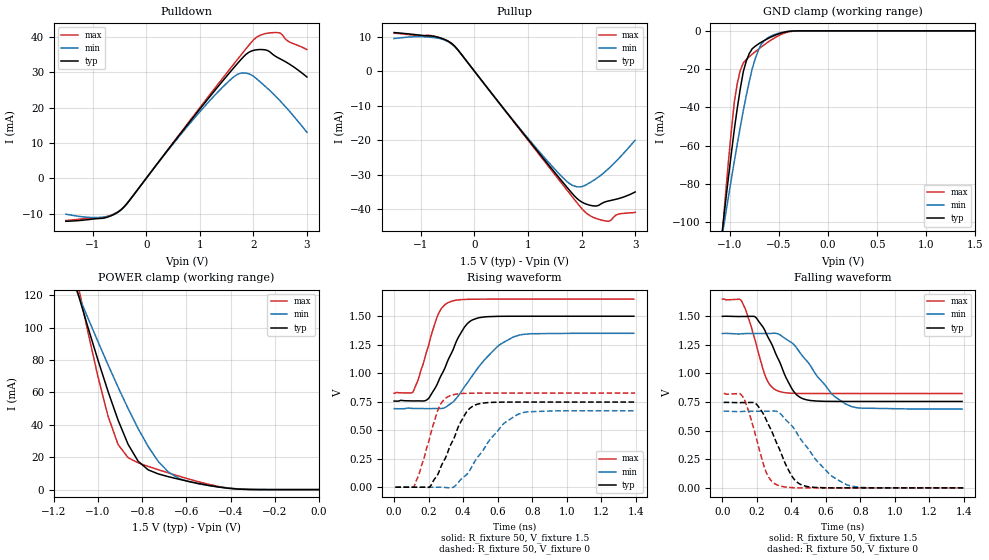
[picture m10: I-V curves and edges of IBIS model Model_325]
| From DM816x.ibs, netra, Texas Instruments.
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| Model based on original model for BSHTLTCSCDDVGPBFZ
|   Sub model SLOWEST_8MA_10PER_N_1P5
[model]   Model_325
|[Description]  1.5V-3-STATE-X-SLOWEST, 8MA, +-10%
|[Input Load]
|[Output Drive] SLOWEST, 8MA
|Voltage   1.5V
|Mode   3-STATE
Model_type   3-state
Polarity   Non-Inverting
Enable   Active-Low
Cref =  15.0000pF
Rref =  100.0000M
Vref =  0V
Vmeas =  0.75
C_comp   1.5249p   1.4275p   1.6205p
[Model Spec]
[Temperature Range]   25   125   -40
[Voltage Range]   1.5   1.35   1.65
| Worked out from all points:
|   slope of the pulldown table from 0 to 0.225 V, typ, clamps not added: 50.1 ohm
|   slope of the pullup table from 0 to 0.225 V, typ, clamps not added: 50.1 ohm
|   GND clamp passes 1 mA (typ) near -0.47 V on its own axis
|   POWER clamp passes 1 mA (typ) near -0.42 V on its own axis
|   rising waveform, R_fixture 50, V_fixture 1.5: 20-80 % time 136ps typ, 207ps min, 98.7ps max; typ from 0.756 V to 1.5 V
|   rising waveform, R_fixture 50, V_fixture 0: 20-80 % time 132ps typ, 190ps min, 95.7ps max; typ from 0 V to 0.747 V
|   falling waveform, R_fixture 50, V_fixture 1.5: 20-80 % time 135ps typ, 201ps min, 95ps max; typ from 1.5 V to 0.755 V
|   falling waveform, R_fixture 50, V_fixture 0: 20-80 % time 132ps typ, 206ps min, 92.7ps max; typ from 0.746 V to 0 V
[POWER_clamp]
-1.5V     321.6mA    260.6mA    415.8mA
-1.091V   121.1mA    120.8mA    126.6mA
-1.076V   114.1mA    115.8mA    116.8mA
-1V       79.88mA    91.3mA     69.56mA
-954.5mV  60.58mA    77.05mA    45.34mA
-909.1mV  42.84mA    63.2mA     27.8mA
-818.2mV  17.47mA    37.6mA     16.51mA
-772.7mV  12.19mA    26.53mA    14.33mA
-681.8mV  7.985mA    10.89mA    10.33mA
-590.9mV  5.092mA    4.952mA    6.596mA
-363.6mV  298.9uA    465.6uA    298.1uA
0V        1.518nA    23.05nA    396.5pA
[Pulldown]
-1.5V     -12.15mA   -10.14mA   -11.93mA
-772.7mV  -11.18mA   -10.9mA    -10.98mA
-590.9mV  -10.12mA   -10.11mA   -9.968mA
-409.1mV  -8.017mA   -7.951mA   -8.019mA
954.5mV   18.69mA    17.99mA    19.06mA
1.455V    28.01mA    26.18mA    28.82mA
1.727V    32.86mA    29.54mA    34.05mA
2V        36.15mA    28.87mA    39.08mA
2.318V    35.62mA    24.67mA    41.12mA
2.5V      33.77mA    21.88mA    41.05mA
2.636V    32.63mA    19.61mA    38.86mA
3V        28.64mA    13.01mA    36.37mA
[Pullup]
-1.5V     11.21mA    9.48mA     11.04mA
-772.7mV  10.17mA    9.762mA    10.21mA
-409.1mV  7.827mA    7.7mA      7.892mA
1.227V    -24.14mA   -23.61mA   -24.51mA
1.682V    -32.78mA   -31.32mA   -33.54mA
1.864V    -36.09mA   -33.28mA   -37.13mA
2V        -37.87mA   -33.46mA   -39.75mA
2.182V    -38.93mA   -32.03mA   -42.07mA
2.409V    -38.05mA   -29.51mA   -43.28mA
2.545V    -37.45mA   -27.6mA    -43.23mA
2.682V    -36.95mA   -25.48mA   -41.44mA
3V        -34.98mA   -19.98mA   -40.92mA
[GND_clamp]
-1.5V     -310mA     -250.5mA   -402.4mA
-1.076V   -103.5mA   -106.1mA   -105.2mA
-1.045V   -89.74mA   -96.32mA   -85.93mA
-954.5mV  -51.19mA   -67.85mA   -36.85mA
-924.2mV  -40.06mA   -58.84mA   -27.27mA
-863.6mV  -21.23mA   -41.55mA   -16.73mA
-833.3mV  -15.79mA   -33.74mA   -15.03mA
-772.7mV  -9.342mA   -19.74mA   -12.19mA
-712.1mV  -6.927mA   -10.35mA   -9.702mA
-621.2mV  -4.26mA    -3.894mA   -6.224mA
-409.1mV  -336.9uA   -288.9uA   -618.6uA
1.5V      1.518nA    2.298uA    269.6pA
[Ramp]
dV/dt_f   0.595976/0.19471469n   0.530056/0.3081009n   0.660776/0.14086159n
dV/dt_r 0.60131872/0.19239325n 0.54085904/0.29503786n  0.6623848/0.14048033n
R_load = 50
[Rising Waveform]
R_fixture = 50
V_fixture = 1.5
V_fixture_min = 1.35
V_fixture_max = 1.65
0s        755.8mV    689.5mV    824.8mV
109.8ps   756.7mV    691mV      837.5mV
200.7ps   780.8mV    689.6mV    1.249V
254.9ps   922.3mV    690.2mV    1.515V
316.3ps   1.128V     721mV      1.622V
371.4ps   1.313V     800.6mV    1.643V
440ps     1.455V     950.7mV    1.649V
595.6ps   1.499V     1.23V      1.65V
702.6ps   1.5V       1.325V     1.65V
1.389ns   1.5V       1.35V      1.65V
[Rising Waveform]
R_fixture = 50
V_fixture = 0
V_fixture_min = 0
V_fixture_max = 0
7.44ps    0V         0V         0V
116.1ps   0V         2.018mV    8.764mV
206ps     0V         0V         429.3mV
260.1ps   135.9mV    0V         700.8mV
322.3ps   354.4mV    -5.463mV   801.4mV
412.3ps   642.8mV    100.9mV    823.4mV
458.6ps   713.4mV    203.8mV    825.1mV
624.2ps   746.4mV    540.7mV    825.9mV
725.6ps   747.1mV    644.4mV    826mV
1.396ns   747.2mV    670.5mV    826mV
[Falling Waveform]
R_fixture = 50
V_fixture = 1.5
V_fixture_min = 1.35
V_fixture_max = 1.65
0s        1.499V     1.349V     1.649V
112.9ps   1.498V     1.347V     1.628V
189.8ps   1.494V     1.349V     1.29V
248.6ps   1.368V     1.349V     979.4mV
319.1ps   1.14V      1.347V     848.5mV
403.7ps   864.5mV    1.266V     826.9mV
456.2ps   786.4mV    1.168V     824.9mV
637.3ps   755.6mV    816mV      824.2mV
749.9ps   755.2mV    709.4mV    824.2mV
1.389ns   755.1mV    688.5mV    824.1mV
[Falling Waveform]
R_fixture = 50
V_fixture = 0
V_fixture_min = 0
V_fixture_max = 0
7.44ps    746.4mV    670.2mV    825.4mV
122.2ps   745.3mV    668.2mV    787.1mV
189.8ps   741.2mV    669.1mV    474.4mV
251.6ps   602.9mV    669.3mV    145.9mV
321.4ps   369.3mV    664.5mV    22.39mV
394ps     125.5mV    555.6mV    3.561mV
443.7ps   37.83mV    447.9mV    0V
615.9ps   0V         127.6mV    0V
726.6ps   0V         23.76mV    0V
1.396ns   0V         0V         0V
